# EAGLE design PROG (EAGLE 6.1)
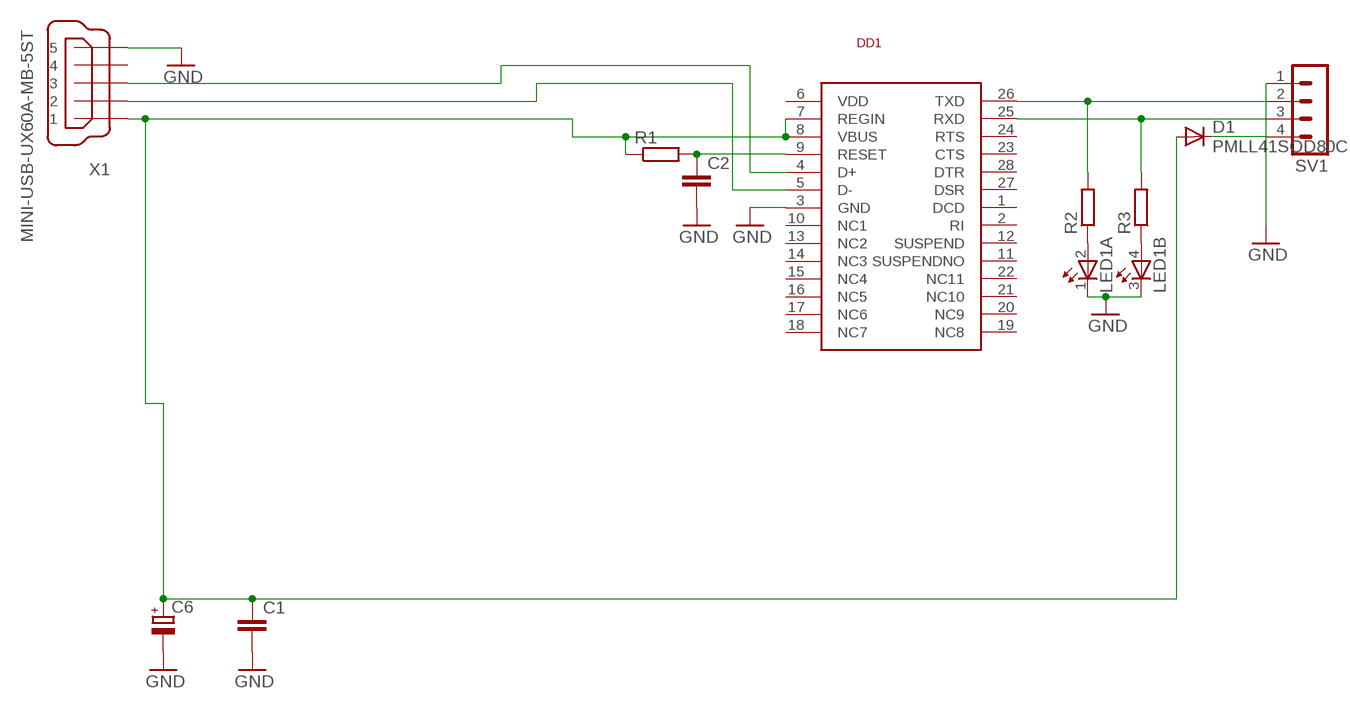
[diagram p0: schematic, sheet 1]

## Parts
C1  C-EUC0402  [C0402]
C2  C-EUC0402  [C0402]
C6  CPOL-EUA/3216-18R  [A/3216-18R]
D1  PMLL41SOD80C  [SOD80C]
DD1  CP2102  [QFN-28]
LED1  TOPLED-2-/  [P-LCC-4/2]
R1  R-EU_M2012  [M2012]
R2  R-EU_M2012  [M2012]
R3  R-EU_M2012  [M2012]
SV1  MA04-1  [MA04-1]
X1  MINI-USB-UX60A-MB-5ST  [UX60A-MB-5ST]

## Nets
GND: C1.2 C2.2 C6.- DD1.3(GND) LED1.1(A:C) LED1.3(B:C) SV1.1 X1.5
N$1: D1.C SV1.4
N$2: DD1.26(TXD) R2.2 SV1.2
N$3: DD1.25(RXD) R3.2 SV1.3
N$4: C1.1 C6.+ D1.A DD1.7(REGIN) DD1.8(VBUS) R1.1 X1.1
N$7: C2.1 DD1.9(RESET) R1.2
N$8: DD1.5(D-) X1.2
N$9: DD1.4(D+) X1.3
N$10: LED1.2(A:A) R2.1
N$11: LED1.4(B:A) R3.1
Unconnected: DD1.1(DCD) DD1.2(RI) DD1.6(VDD) DD1.10(NC1) DD1.11(SUSPENDNO) DD1.12(SUSPEND) DD1.13(NC2) DD1.14(NC3) DD1.15(NC4) DD1.16(NC5) DD1.17(NC6) DD1.18(NC7) DD1.19(NC8) DD1.20(NC9) DD1.21(NC10) DD1.22(NC11) DD1.23(CTS) DD1.24(RTS) DD1.27(DSR) DD1.28(DTR) X1.4

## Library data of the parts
C1 C2 = resistor:C-EU: CAPACITOR, European symbol
C6 = resistor:CPOL-EU: POLARIZED CAPACITOR, European symbol
D1 = diode:PMLL41*: High-speed diodes
DD1 = pepelac:CP2102
LED1 = led:TOPLED-2-: Multi TOPLED® (two color) LG T672, LP T672 LSY T67B LSW T67C LSY T675 LSY T676 LSG T677 LSG T770 Source: http://www.osram.convergy.de/
R1-R3 = resistor:R-EU_: RESISTOR, European symbol
SV1 = con-lstb:MA04-1: PIN HEADER; OC_FARNELL: unknown; OC_NEWARK: unknown
X1 = con-hirose:MINI-USB-: MINI USB Connector Source: http://www.hirose.co.jp/cataloge_hp/e24000019.pdf; OC_FARNELL: unknown; OC_NEWARK: unknown

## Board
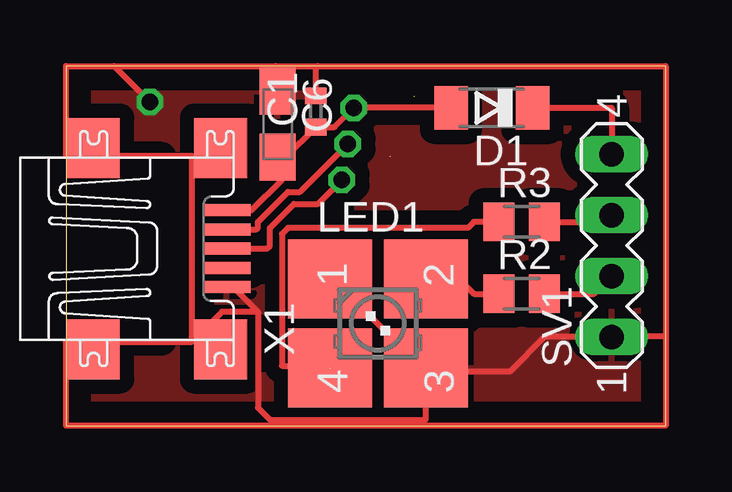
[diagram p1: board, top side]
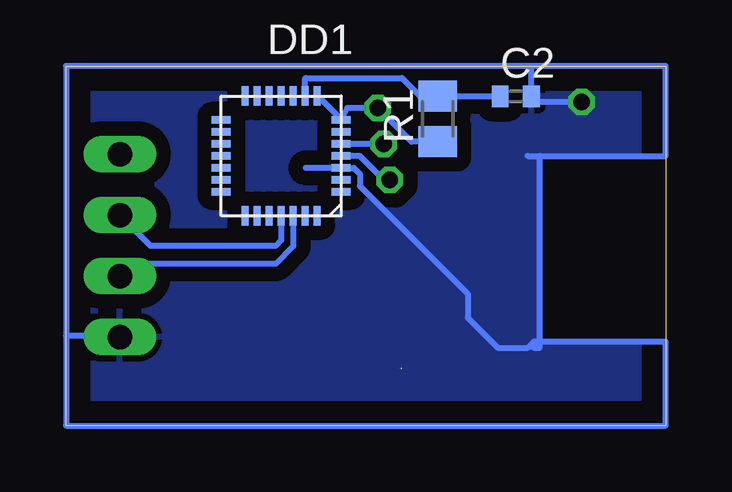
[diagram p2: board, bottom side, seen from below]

Size 25 x 15 mm. Coordinates in mm from the lower left corner, seen from the top.
Outline: 0,0 25,0 25,15 0,15 0,0
Copper layers (1*16): Top 0.035mm / dielectric 1.5mm / Bottom 0.035mm
Design rules: minimum track width 10mil, minimum drill 24mil, track to track 8mil, track to pad 8mil, pad to pad 8mil, via to via 8mil, smd to smd 8mil, copper to edge 40mil, drill to drill 8mil, minimum pad ring 10mil, minimum via ring 8mil, stop-mask expansion 4mil, vias tented up to drill 0mil, thermal gap 10mil

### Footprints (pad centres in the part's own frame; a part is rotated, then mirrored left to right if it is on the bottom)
C0402 = smd 0.7 x 0.9: 1 -0.65,0; 2 0.65,0
A/3216-18R = smd 1.95 x 1.5: + 1.375,0; - -1.375,0
SOD80C = smd 1.4 x 1.8: A 1.7,0; C -1.7,0
QFN-28 = smd 0.8 x 0.3: 1 -2.5,1.5; 2 -2.5,1; 3 -2.5,0.5; 4 -2.5,0; 5 -2.5,-0.5; 6 -2.5,-1; 7 -2.5,-1.5; 15 2.5,-1.5; 16 2.5,-1; 17 2.5,-0.5; 18 2.5,0; 19 2.5,0.5; 20 2.5,1; 21 2.5,1.5 | smd 0.3 x 0.8: 8 -1.5,-2.5; 9 -1,-2.5; 10 -0.5,-2.5; 11 0,-2.5; 12 0.5,-2.5; 13 1,-2.5; 14 1.5,-2.5; 22 1.5,2.5; 23 1,2.5; 24 0.5,2.5; 25 0,2.5; 26 -0.5,2.5; 27 -1,2.5; 28 -1.5,2.5
P-LCC-4/2 = smd 3.3 x 3.5: 1 -1.85,-2; 2 -1.85,2; 3 1.85,2; 4 1.85,-2
M2012 = smd 1.3 x 1.6: 1 -0.95,0; 2 0.95,0
MA04-1 = drill 1.016 long: 1 -3.81,0; 2 -1.27,0; 3 1.27,0; 4 3.81,0
UX60A-MB-5ST = smd 2 x 0.5: 1 2.25,1.6; 2 2.25,0.8; 3 2.25,0; 4 2.25,-0.8; 5 2.25,-1.6 | smd 2.2 x 2.5: M1 -3.3,-4.2; M2 -3.3,4.2; M3 2,4.2; M4 2,-4.2

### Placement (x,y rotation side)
C1  10.42,13.1 90 top
C2  6.25,13.73 0 bottom
C6  8.83,12.57 270 top
D1  17.76,13.25 180 top
DD1  16.03,11.25 180 bottom
LED1  13,4.26 270 top
R1  9.5,12.79 90 bottom
R2  19,5.5 0 top
R3  19,8.5 0 top
SV1  22.75,7.5 90 top
X1  4.45,7.38 0 top

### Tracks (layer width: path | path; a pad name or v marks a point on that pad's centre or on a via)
GND  (via drill 0.7)
  Top 0.25: SV1.1 19.94,3.69 18.5,2.25 15.17,2.25 LED1.3 | LED1.3 14.84,2.41 11.75,5.5 11.62,5.5 LED1.1 | X1.5 6.97,5.78 8,4.75 | 8,4.75 8,0.75 8.5,0.25 15,0.25 LED1.3 | 2,15 8.75,15 | 8.75,15 10.5,15 | 10.5,15 25,15 25,3.75 | 25,3.75 25,0 0,0 0,3.5 5.25,3.5 | 5.25,3.5 5.25,11.25 0,11.25 0,15 2,15 | 8,4.75 6.5,4.75 5.25,3.5 | 22.75,3.75 25,3.75 | C6.- 8.83,14.92 8.75,15 | C1.2 10.42,14.92 10.5,15 | 2,15 v3.5,13.5
  Bottom 0.25: DD1.3 13,10.75 12.75,10.5 12.75,10 8.25,5.5 8.25,4.5 7,3.25 5.75,3.25 5.5,3.5 | 5.75,11.25 5.25,11.25 | 5.25,11.25 0,11.25 0,15 5.75,15 | 5.75,15 25,15 25,3.75 | 25,3.75 25,0 0,0 0,3.5 5.5,3.5 | 5.5,3.5 5.5,3.25 5.25,3.25 5.25,11.25 | C2.2 5.6,14.85 5.75,15 | 22.75,3.75 25,3.75 | v3.5,13.5 5.25,13.5 5.5,13.75
  pour Bottom (isolate 0.6): 0,15 25,15 25,0 0,0 0,0.25 0,3.5 5.25,3.5 5.25,11.25 0,11.25
  pour Top (isolate 0.6): 0,15 25,15 25,0 0,0 0,3.5 5.25,3.5 5.25,11.25 0,11.25
N$1
  Top 0.25: D1.C 22.75,13.25 SV1.4
N$2
  Top 0.25: R2.2 22.02,5.5 SV1.2
  Bottom 0.25: DD1.26 15.53,7.47 16.25,6.75 22.23,6.75 SV1.2
N$3
  Top 0.25: R3.2 22.48,8.5 SV1.3
  Bottom 0.25: DD1.25 16.03,7.72 16.25,7.5 21.48,7.5 SV1.3
N$4  (via drill 0.7)  (1 unrouted)
  Top 0.25: X1.1 7.73,8.98 9,10.25 9,11.03 C6.+ 9.16,11.2 C1.1 11.2,12.45 v12,13.25 D1.A
  Bottom 0.25: 14.5,13.75 13.53,12.78 DD1.7 13.27,13.25 v12,13.25 10.59,11.84 R1.1
N$5
  Bottom 0.25: 13.5,10.75 15,10.75
N$7
  Bottom 0.25: DD1.9 15.03,14.47 15,14.5 11,14.5 10.25,13.75 R1.2 C2.1
N$8  (via drill 0.7)
  Top 0.25: X1.2 7.93,8.18 8,8.25 8,8.5 9.25,9.75 9.75,9.75 v11.75,11.75
  Bottom 0.25: v11.75,11.75 DD1.5
N$9  (via drill 0.7)  (1 unrouted)
  Top 0.25: X1.3 8.38,7.38 8.5,7.5 8.5,8.25 9.5,9.25 10.5,9.25 v11.5,10.25
  Bottom 0.25: v11.5,10.25 11.75,10.25 12.75,11.25 13.5,11.25
N$10
  Top 0.25: LED1.2 16.39,6.11 17,5.5 R2.1
N$11  (1 unrouted)
  Top 0.25: R3.1 17,8.5 16.75,8.25 9.25,8.25 9,8 9,2.5 11,2.5 11,2.36 | 11,2.36 11.02,2.36 11.02,2.27 11,2.25 11,2.36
